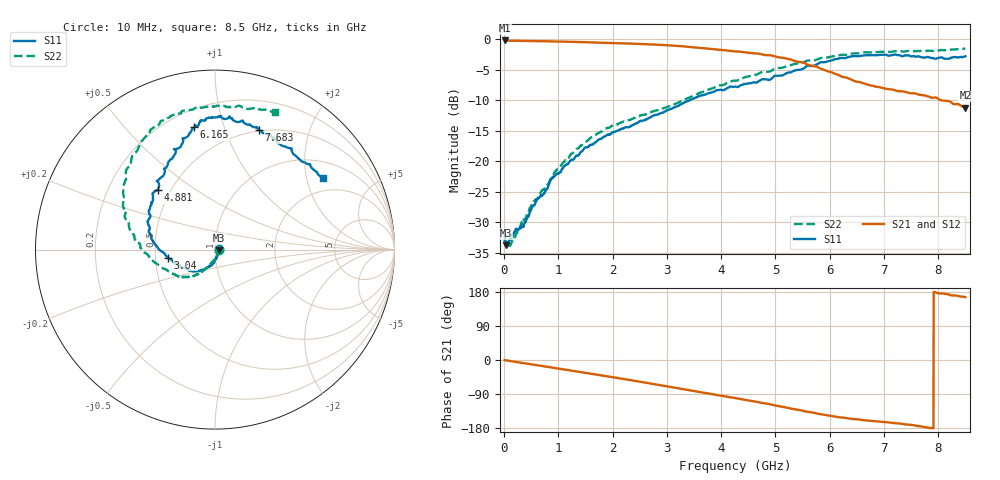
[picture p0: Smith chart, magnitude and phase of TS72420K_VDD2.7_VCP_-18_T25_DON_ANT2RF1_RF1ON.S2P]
!Agilent Technologies,E5071C,MY46417908,A.11.23
!Date: Thu Oct 03 16:40:33 2019
!Data & Calibration Information:
!Freq	S11:SOLT2(ON)	S21:SOLT2(ON)	S12:SOLT2(ON)	S22:SOLT2(ON)
!PortZ  Port1:50+j0  Port2:50+j0
!Above PortZ is port z conversion or system Z0 setting when saving the data.
!When reading, reference impedance value at option line is always used.
# Hz S dB R 50
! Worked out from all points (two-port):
!   1601 points, 10 MHz to 8.5 GHz, reference 50 ohm
!   highest |S21| = -0.24 dB at 10 MHz (marker M1); lowest = -11.2 dB at 8.5 GHz (marker M2)
!   |S21| within 3 dB of the highest: start of sweep to 5.218 GHz
!   lowest |S11| = -33.8 dB at 31.23 MHz (marker M3), VSWR 1.04, Z = 52.1 - j0.373 ohm
!   |S11| at or under -10 dB: start of sweep to 3.432 GHz
!   |S22| runs from -33.9 to -1.6 dB; largest |S21 - S12| = 0.0051
!   S11 on the Smith chart (normalised r, x): 10 MHz: 1.05, +0.01; 3.04 GHz: 0.58, -0.06; 4.881 GHz: 0.42, +0.36; 6.165 GHz: 0.30, +0.80; 7.683 GHz: 0.49, +1.32; 8.5 GHz: 1.49, +2.50
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1e7  -32.59 8.7  -0.24 -0.3  -0.25 -0.3  -33.28 -11.1
3.1225e7  -33.78 -10.1  -0.26 -0.8  -0.27 -0.8  -33.51 -16.1
1.320438e8  -32.84 -23.8  -0.29 -3.1  -0.29 -3.1  -33.43 -35.2
3.602125e8  -30.75 -57.3  -0.32 -8.3  -0.32 -8.3  -29.56 -63.8
5.512375e8  -27.22 -76.9  -0.36 -12.5  -0.36 -12.5  -26.64 -85.5
7.634875e8  -24.72 -89.9  -0.38 -17.3  -0.38 -17.2  -24.30 -94.9
8.855312e8  -22.71 -94.2  -0.41 -20.0  -0.41 -19.9  -22.40 -105.5
1.426769e9  -18.43 -116.5  -0.52 -32.2  -0.51 -32.2  -17.43 -119.5
1.893719e9  -15.75 -132.6  -0.63 -42.9  -0.62 -42.9  -14.58 -128.0
2.843538e9  -12.33 -163.9  -0.95 -65.6  -0.95 -65.6  -11.63 -147.8
3.039869e9  -11.53 -170.3  -1.05 -70.4  -1.05 -70.4  -11.01 -153.7
3.634169e9  -9.25 173.3  -1.47 -85.1  -1.49 -85.1  -8.73 -172.3
4.255e9  -7.81 155.3  -2.04 -100.3  -2.05 -100.1  -6.84 170.6
4.881138e9  -6.72 133.9  -2.65 -116.3  -2.68 -116.2  -5.34 156.3
5.289719e9  -5.43 120.1  -3.39 -128.3  -3.40 -128.4  -4.27 146.2
5.671769e9  -4.44 110.2  -4.41 -138.4  -4.40 -138.3  -3.54 135.0
6.16525e9  -3.20 99.7  -5.92 -150.9  -5.96 -151.0  -2.67 122.3
6.664038e9  -2.66 93.0  -7.39 -159.3  -7.46 -159.3  -2.18 112.7
7.088538e9  -2.74 85.8  -8.21 -164.9  -8.24 -164.8  -2.11 104.9
7.682838e9  -2.98 69.7  -9.16 -175.1  -9.06 -175.3  -1.96 91.6
8.255912e9  -3.01 42.4  -10.52 170.2  -10.49 170.3  -1.73 74.1
8.5e9  -2.83 33.8  -11.25 166.0  -11.29 166.1  -1.55 66.5
